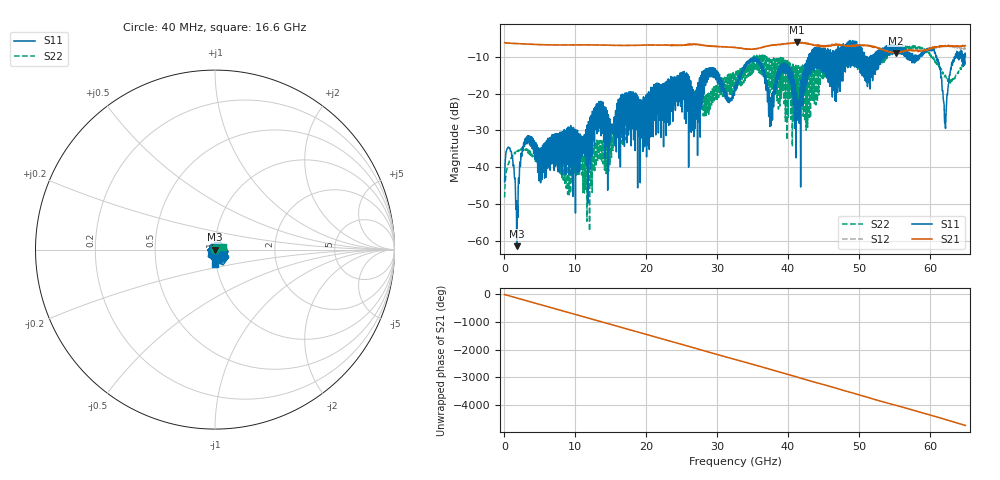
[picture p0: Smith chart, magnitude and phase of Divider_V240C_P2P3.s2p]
! Created Tue Jul 15 20:13:52 2008
# hz S ma R 50
! 2 Port Network Data from blockName block
! freq  magS11  angS11  magS21  angS21  magS12  angS12  magS22  angS22
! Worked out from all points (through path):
!   1601 points, 40 MHz to 65 GHz, reference 50 ohm
!   highest |S21| = -6.05 dB at 41.29 GHz (marker M1); lowest = -8.9 dB at 55.22 GHz (marker M2)
!   group delay of S21, straight-line fit = 202 ps
!   lowest |S11| = -61.5 dB at 1.745 GHz (marker M3), VSWR 1.00, Z = 50 - j0.0822 ohm
!   |S11| at or under -10 dB: start of sweep to 42.97 GHz; 51.12 GHz to 51.48 GHz (362.2 MHz wide, 0.706 % of centre); 60.96 GHz to 63.45 GHz (2.49 GHz wide, 4 % of centre)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
!   |S22| runs from -57.3 to -6.9 dB; largest |S21 - S12| = 0.06
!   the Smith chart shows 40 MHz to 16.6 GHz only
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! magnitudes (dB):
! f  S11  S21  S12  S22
! 40 MHz  -44.0  -6.1  -6.1  -48.2
! 852 MHz  -35.6  -6.3  -6.3  -37.6
! 1.745 GHz  -61.5  -6.3  -6.3  -35.9
! 3.207 GHz  -33.6  -6.5  -6.5  -35.6
! 10.88 GHz  -31.5  -6.7  -6.7  -42.1
! 13.28 GHz  -30.3  -6.7  -6.7  -34.2
! 14.9 GHz  -28.7  -6.8  -6.8  -39.3
! 21.72 GHz  -30.7  -6.8  -6.8  -21.2
! 26.96 GHz  -19.6  -6.6  -6.5  -19.0
! 29.11 GHz  -15.4  -7.0  -7.0  -19.4
! 32.52 GHz  -17.8  -7.4  -7.4  -17.1
! 35.61 GHz  -11.5  -7.7  -7.8  -9.4
! 37.55 GHz  -21.1  -6.8  -6.9  -10.8
! 39.62 GHz  -14.4  -6.4  -6.5  -27.5
! 41.29 GHz  -26.4  -6.0  -6.0  -12.5
! 43.36 GHz  -8.1  -6.6  -6.6  -21.7
! 54.2 GHz  -7.3  -8.5  -8.5  -8.2
! 55.22 GHz  -8.3  -8.9  -8.5  -7.7
! 60.49 GHz  -7.9  -7.5  -7.7  -10.1
! 62.16 GHz  -28.3  -6.9  -6.8  -15.1
! 63.34 GHz  -11.3  -7.0  -7.1  -15.5
! 65 GHz  -9.8  -6.9  -8.0  -11.3
